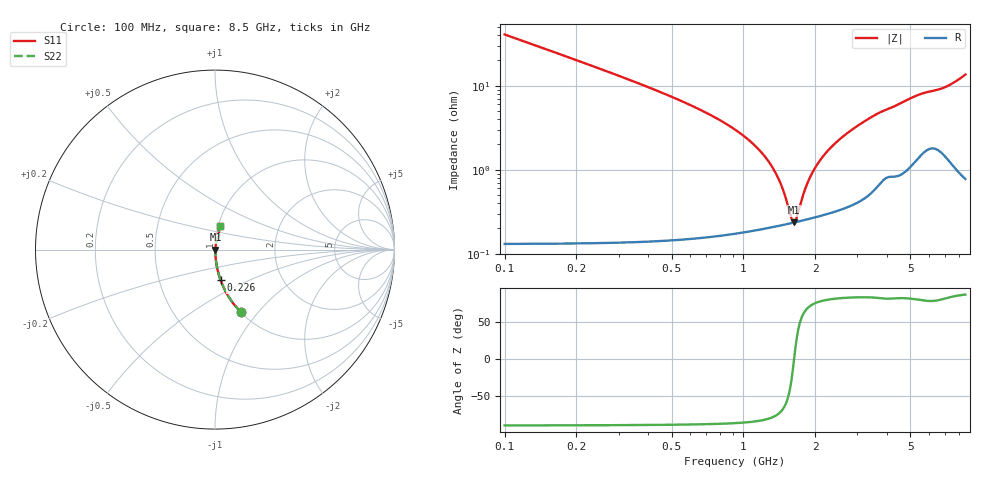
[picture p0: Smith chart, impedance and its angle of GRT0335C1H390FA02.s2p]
!Murata Part Number: GRT0335C1H390FA02
!These Parameters are Measured in Series Mode Connection
!Data Generated on Jun 19, 2026
!  o--ll--o
!Port1  Port2
!  o------o
!Operation Temp=25[degC], DC Bias Voltage=0[V]
!Freq. Start=100[MHz] Stop=9[GHz] 401[Steps]
# Hz S RI R 50
!Freq.(Hz) S11(Real) S11(Imag) S21(Real) S21(Imag) S12(Real) S12(Imag) S22(Real) S22(Imag)
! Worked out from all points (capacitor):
!   401 points, 100 MHz to 8.5 GHz, reference 50 ohm
!   read as one part in series: C = 39 pF near 142 MHz
!   lowest |Z| = 236 mohm at 1.633 GHz (marker M1)
!   series resonance near 1.63 GHz, so ESL is about 240 pH
!   S11 on the Smith chart (normalised r, x): 100 MHz: 1.00, -0.81; 226 MHz: 1.00, -0.35; 8.5 GHz: 1.02, +0.27
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1e8  0.1426 -0.3481  0.8574 0.3481  0.8574 0.3481  0.1426 -0.3481
2.26e8  0.0316 -0.1712  0.9684 0.1712  0.9684 0.1712  0.0316 -0.1712
3.31e8  0.0151 -0.1162  0.9849 0.1162  0.9849 0.1162  0.0151 -0.1162
4.78e8  0.00744 -0.0772  0.9926 0.0772  0.9926 0.0772  0.00744 -0.0772
1.024e9  0.00238 -0.0239  0.9976 0.0239  0.9976 0.0239  0.00238 -0.0239
1.213e9  0.00219 -0.0149  0.9978 0.0149  0.9978 0.0149  0.00219 -0.0149
1.381e9  0.00219 -0.00825  0.9978 0.00825  0.9978 0.00825  0.00219 -0.00825
1.507e9  0.00225 -0.00389  0.9978 0.00389  0.9978 0.00389  0.00225 -0.00389
1.591e9  0.00231 -0.00119  0.9977 0.00119  0.9977 0.00119  0.00231 -0.00119
1.633e9  0.00235 9.69e-05  0.9976 -9.69e-05  0.9976 -9.69e-05  0.00235 9.69e-05
1.675e9  0.00239 0.00136  0.9976 -0.00136  0.9976 -0.00136  0.00239 0.00136
1.78e9  0.00251 0.00438  0.9975 -0.00438  0.9975 -0.00438  0.00251 0.00438
1.864e9  0.00262 0.00668  0.9974 -0.00668  0.9974 -0.00668  0.00262 0.00668
1.969e9  0.00277 0.00943  0.9972 -0.00943  0.9972 -0.00943  0.00277 0.00943
2.074e9  0.00293 0.0121  0.9971 -0.0121  0.9971 -0.0121  0.00293 0.0121
2.41e9  0.00355 0.02  0.9965 -0.02  0.9965 -0.02  0.00355 0.02
2.914e9  0.00482 0.0308  0.9952 -0.0308  0.9952 -0.0308  0.00482 0.0308
3.586e9  0.00794 0.0443  0.9921 -0.0443  0.9921 -0.0443  0.00794 0.0443
4.3e9  0.0113 0.0554  0.9887 -0.0554  0.9887 -0.0554  0.0113 0.0554
5.707e9  0.022 0.0774  0.978 -0.0774  0.978 -0.0774  0.022 0.0774
7.114e9  0.0224 0.0938  0.9776 -0.0938  0.9776 -0.0938  0.0224 0.0938
8.5e9  0.0253 0.1309  0.9747 -0.1309  0.9747 -0.1309  0.0253 0.1309
